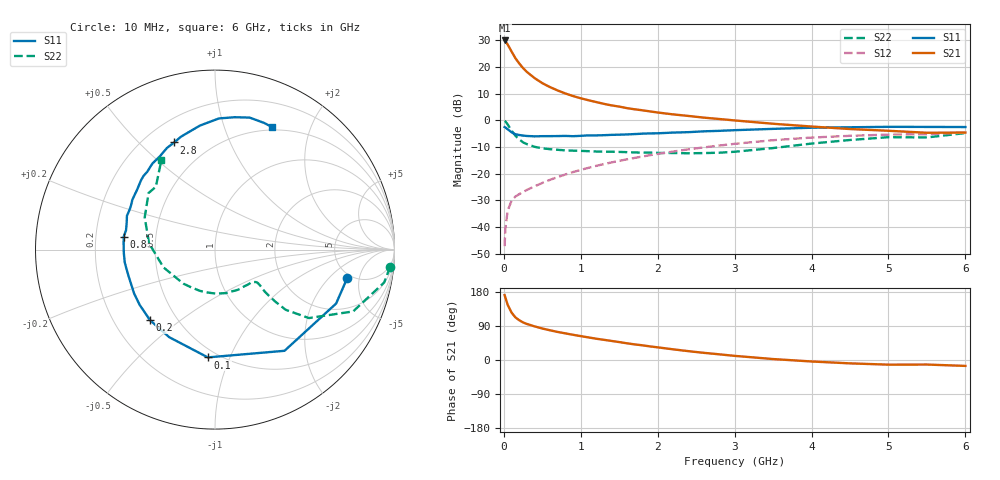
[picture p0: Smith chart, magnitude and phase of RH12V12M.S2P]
! SIEMENS Small Signal Semiconductors
! BFR106
! Si NPN RF Bipolar Junction Transistor in SOT23
! VCE = 12 V  IC = 12 mA
! Common Emitter S-Parameters:  August  1996
# GHz  S  MA  R  50
!  f  S11  S21  S12  S22
! GHz  MAG  ANG  MAG  ANG  MAG  ANG  MAG  ANG
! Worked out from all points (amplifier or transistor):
!   36 points, 10 MHz to 6 GHz, reference 50 ohm
!   highest |S21| = 30.0 dB at 10 MHz (marker M1)
!   |S21| within 3 dB of that: start of sweep to 78.18 MHz
!   unconditionally stable (mu >= 1): 476.2 MHz to 2.028 GHz
!   at 250 MHz: K = 0.74, MSG = 23.2 dB, |S12| = -26.8 dB
!   at 1.4 GHz: K = 1.09, MAG = 8.9 dB, |S12| = -15.7 dB
!   at 6 GHz: K = 0.99, MSG = 0.0 dB, |S12| = -4.5 dB
!   S11 on the Smith chart (normalised r, x): 10 MHz: 4.56, -3.36; 100 MHz: 0.44, -0.83; 200 MHz: 0.36, -0.39; 800 MHz: 0.32, +0.06; 2.8 GHz: 0.32, +0.64; 6 GHz: 0.46, +1.47
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0.01  0.7534 -12.2  31.64 171.3  0.0044 84.9  0.9805 -5.6
0.02  0.7387 -24.0  30.72 164.8  0.0095 75.8  0.9602 -11.0
0.05  0.6841 -55.5  26.5 145.5  0.0203 65.7  0.8433 -24.1
0.1  0.6019 -93.8  19.66 125.2  0.0313 54.0  0.6474 -36.1
0.15  0.5506 -117.6  14.73 112.5  0.0375 49.8  0.5175 -40.4
0.2  0.5344 -132.6  11.73 105.0  0.0415 50.1  0.4425 -40.8
0.25  0.5207 -143.7  9.6 99.1  0.0456 50.6  0.3889 -40.5
0.3  0.5126 -151.6  8.113 95.1  0.0499 52.1  0.3598 -40.1
0.4  0.5038 -163.3  6.22 88.7  0.0583 55.8  0.3208 -38.5
0.5  0.508 -171.9  5.013 83.1  0.0674 58.5  0.3007 -37.9
0.6  0.5084 -178.0  4.223 78.4  0.0771 60.5  0.2895 -38.6
0.8  0.5137 171.9  3.207 70.3  0.0971 62.9  0.2749 -41.2
0.9  0.5073 167.7  2.868 66.5  0.1079 63.7  0.2718 -42.8
1.1  0.5256 159.0  2.396 59.6  0.1295 64.3  0.2656 -48.3
1.3  0.5296 151.8  2.05 53.3  0.1522 63.8  0.2602 -53.7
1.6  0.5475 142.4  1.704 44.1  0.1869 62.3  0.2546 -63.9
2.2  0.5928 126.1  1.301 28.2  0.2614 57.2  0.2454 -89.0
2.8  0.6389 110.9  1.066 15.0  0.3385 49.6  0.2487 -122.3
3.5  0.6962 96.9  0.868 2.5  0.4268 39.0  0.304 -161.1
4.5  0.7458 81.5  0.691 -8.9  0.5155 21.9  0.4306 155.4
5.5  0.757 68.9  0.588 -12.0  0.5522 9.8  0.4806 133.3
6  0.7532 65.0  0.594 -15.6  0.593 1.8  0.5805 121.0
